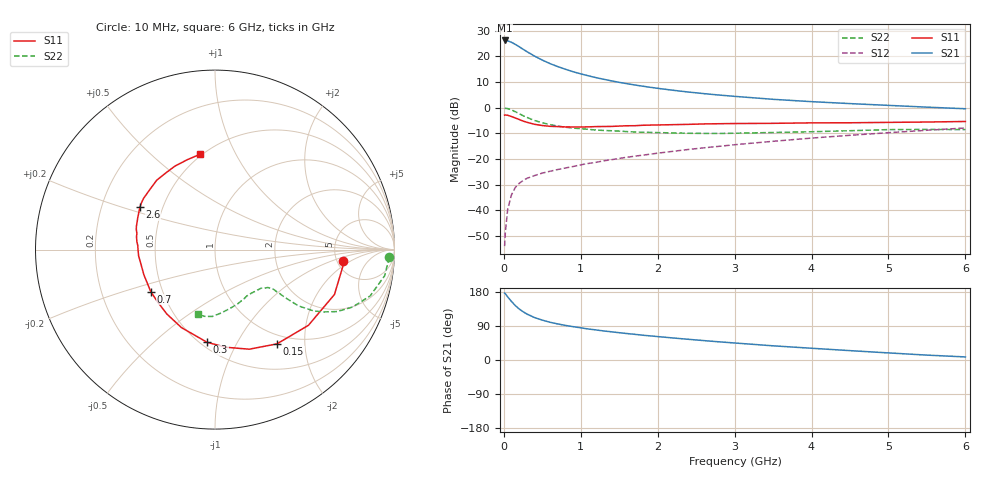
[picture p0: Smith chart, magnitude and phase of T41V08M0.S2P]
! Infineon Technologies  Discrete & RF Semiconductors
! BFR182T
! Si NPN RF Bipolar Junction Transistor in SC75
! VCE = 1 V  IC = 8 mA
! Common Emitter S-Parameters:  October  1999
# GHz  S  MA  R  50
!  f  S11  S21  S12  S22
! GHz  MAG  ANG  MAG  ANG  MAG  ANG  MAG  ANG
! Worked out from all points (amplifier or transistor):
!   36 points, 10 MHz to 6 GHz, reference 50 ohm
!   highest |S21| = 26.2 dB at 10 MHz (marker M1)
!   |S21| within 3 dB of that: start of sweep to 228.4 MHz
!   unconditionally stable (mu >= 1): 931.2 MHz to 4.204 GHz
!   at 250 MHz: K = 0.42, MSG = 25.6 dB, |S12| = -28.4 dB
!   at 1.4 GHz: K = 1.12, MAG = 13.3 dB, |S12| = -20.3 dB
!   at 6 GHz: K = 0.89, MSG = 3.7 dB, |S12| = -7.9 dB
!   S11 on the Smith chart (normalised r, x): 10 MHz: 5.57, -1.50; 150 MHz: 0.86, -1.49; 300 MHz: 0.54, -0.76; 700 MHz: 0.43, -0.25; 2.6 GHz: 0.37, +0.23; 6 GHz: 0.49, +0.73
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0.01  0.7136 -5.3  20.35 176.6  0.002 81.5  0.969 -2.5
0.02  0.7197 -6.9  20.29 174.9  0.0038 93.5  0.9683 -3.5
0.05  0.711 -20.6  20.02 166.5  0.0105 83.2  0.9563 -8.8
0.1  0.67 -39.0  18.7 154.4  0.0201 72.5  0.9022 -16.6
0.15  0.6285 -56.7  17.04 143.4  0.028 66.2  0.8316 -22.6
0.2  0.5869 -71.0  15.36 134.6  0.0335 61.9  0.7631 -26.9
0.25  0.5476 -83.6  13.72 127.4  0.0379 58.0  0.6967 -29.9
0.3  0.5184 -94.9  12.31 121.3  0.0419 55.5  0.6455 -31.9
0.4  0.473 -113.3  10.08 111.9  0.0475 53.7  0.5601 -34.0
0.5  0.448 -126.8  8.44 105.2  0.053 53.5  0.5065 -34.2
0.6  0.4324 -138.0  7.209 99.6  0.0576 53.7  0.467 -34.4
0.7  0.4277 -146.8  6.307 95.2  0.0622 54.7  0.4373 -34.2
0.9  0.4204 -160.7  5.009 88.0  0.0712 56.6  0.399 -34.2
1.1  0.4221 -171.3  4.162 81.8  0.0818 58.6  0.377 -34.9
1.3  0.4288 -179.7  3.564 76.6  0.0922 60.0  0.3591 -36.1
1.6  0.4434 170.5  2.926 69.8  0.108 61.4  0.3412 -38.6
2.2  0.4658 157.5  2.178 58.1  0.141 62.7  0.3219 -46.5
2.6  0.4812 150.4  1.874 51.2  0.1648 62.6  0.3147 -52.6
3.5  0.4944 136.7  1.452 37.4  0.2209 60.5  0.3278 -67.5
4.5  0.507 123.3  1.198 24.7  0.2891 55.7  0.355 -84.5
5.5  0.5242 107.0  1.022 12.9  0.3624 49.7  0.3763 -98.9
6  0.5372 99.1  0.951 8.1  0.4011 45.8  0.3732 -105.1
